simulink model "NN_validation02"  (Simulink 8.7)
settings: Solver=ode45  StartTime=0.0  StopTime=2000  RelTol=1e-3
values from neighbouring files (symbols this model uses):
  Ts = 0.2    [init_model.m]
libraries: neural x26

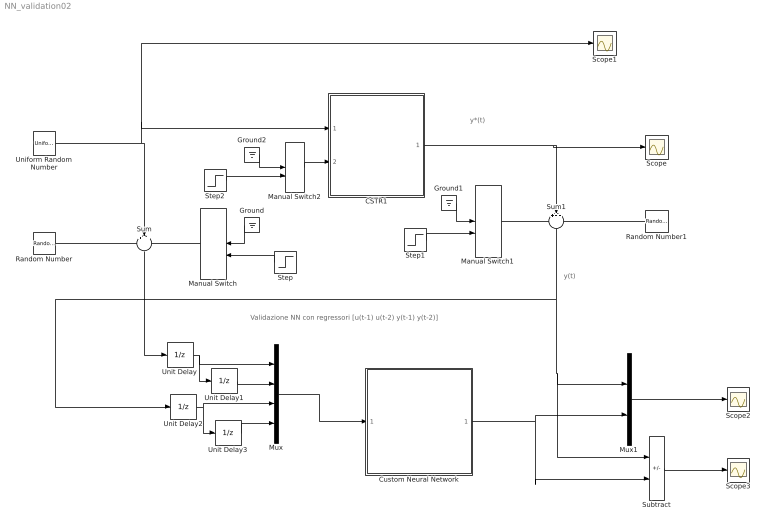
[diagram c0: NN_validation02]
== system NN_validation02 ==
  note: y(t)
  note: y*(t)
  note: Validazione NN con regressori [u(t-1) u(t-2) y(t-1) y(t-2)]
  CSTR1 : Subsystem
  Custom Neural Network : Subsystem
  Ground : Ground
  Ground1 : Ground
  Ground2 : Ground
  Manual Switch : ManualSwitch
  Manual Switch1 : ManualSwitch
  Manual Switch2 : ManualSwitch
  Mux : Mux
  Mux1 : Mux  Inputs=2
  Random Number : RandomNumber  Variance=0.0001  Seed=1  SampleTime=Ts
  Random Number1 : RandomNumber  Variance=0.0005  Seed=2  SampleTime=Ts
  Scope{,1..3} (4 alike) : Scope
  Step : Step  Time=1000  After=10  SampleTime=0
  Step1 : Step  Time=1000  After=10  SampleTime=0
  Step2 : Step  Time=1000  SampleTime=0
  Subtract : Sum  Inputs=+-
  Sum : Sum  Inputs=+++  SaturateOnIntegerOverflow=on
  Sum1 : Sum  Inputs=+++  SaturateOnIntegerOverflow=on
  Uniform Random Number : UniformRandomNumber  Minimum=0  Maximum=4  SampleTime=20
  Unit Delay{,1..3} (4 alike) : UnitDelay  SampleTime=Ts  HasFrameUpgradeWarning=on
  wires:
  Uniform Random Number/1 -> CSTR1/1(w), Scope1/1, Sum/2
  Random Number/1 -> Sum/1
  Manual Switch/1 -> Sum/3
  Sum/1 -> Unit Delay/1
  Ground/1 -> Manual Switch/1
  Step/1 -> Manual Switch/2
  Ground1/1 -> Manual Switch1/1
  Step1/1 -> Manual Switch1/2
  CSTR1/1(Cb) -> Scope/1, Sum1/2
  Manual Switch1/1 -> Sum1/1
  Random Number1/1 -> Sum1/3
  Unit Delay/1 -> Unit Delay1/1, Mux/1
  Unit Delay1/1 -> Mux/2
  Unit Delay2/1 -> Mux/3, Unit Delay3/1
  Unit Delay3/1 -> Mux/4
  Mux/1 -> Custom Neural Network/1(Input)
  Step2/1 -> Manual Switch2/2
  Manual Switch2/1 -> CSTR1/2(f)
  Ground2/1 -> Manual Switch2/1
  Subtract/1 -> Scope3/1
  Mux1/1 -> Scope2/1
  Sum1/1 -> Mux1/1, Subtract/1, Unit Delay2/1
  Custom Neural Network/1(Output) -> Subtract/2, Mux1/2

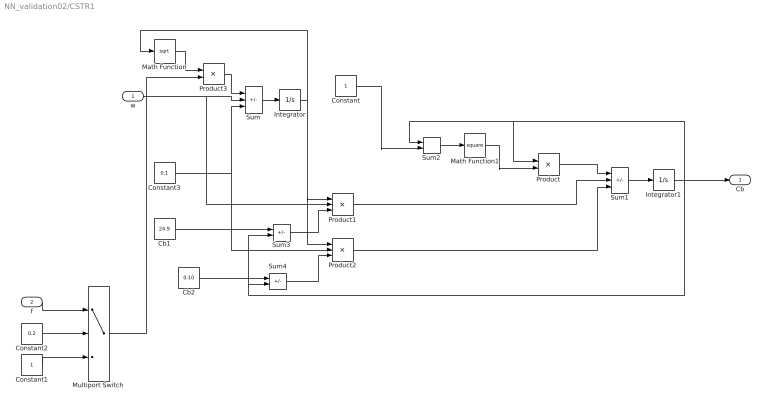
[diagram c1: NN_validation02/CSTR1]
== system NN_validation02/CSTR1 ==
  w : Inport
  f : Inport  Port=2
  Cb1 : Constant  Value=24.9
  Cb2 : Constant  Value=0.10
  Constant : Constant
  Constant1 : Constant
  Constant2 : Constant  Value=0.2
  Constant3 : Constant  Value=0.1
  Integrator : Integrator  InitialCondition=30  LimitOutput=on  LowerSaturationLimit=1
  Integrator1 : Integrator  InitialCondition=22
  Math Function : Math  Operator=sqrt
  Math Function1 : Math  Operator=square
  Multiport Switch : MultiPortSwitch  DataPortOrder=Zero-based contiguous  Inputs=2  zeroidx=on
  Product : Product  Inputs=*/  SaturateOnIntegerOverflow=on
  Product1 : Product  Inputs=/**  SaturateOnIntegerOverflow=on
  Product2 : Product  Inputs=/**  SaturateOnIntegerOverflow=on
  Product3 : Product
  Sum : Sum  Inputs=-++  SaturateOnIntegerOverflow=on
  Sum1 : Sum  Inputs=-++  SaturateOnIntegerOverflow=on
  Sum2 : Sum  SaturateOnIntegerOverflow=on
  Sum3 : Sum  Inputs=+-  SaturateOnIntegerOverflow=on
  Sum4 : Sum  Inputs=+-  SaturateOnIntegerOverflow=on
  Cb : Outport
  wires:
  Sum/1 -> Integrator/1
  Product3/1 -> Sum/1
  Math Function/1 -> Product3/1
  Integrator/1 -> Math Function/1, Product1/1, Product2/1
  Sum3/1 -> Product1/3
  Sum4/1 -> Product2/3
  Sum2/1 -> Math Function1/1
  Sum1/1 -> Integrator1/1
  Math Function1/1 -> Product/2
  Product/1 -> Sum1/1
  Product1/1 -> Sum1/2
  Product2/1 -> Sum1/3
  w/1 -> Sum/2, Product1/2
  Constant3/1 -> Product2/2, Sum/3
  Integrator1/1 -> Sum3/2, Sum4/2, Sum2/1, Product/1, Cb/1
  Constant1/1 -> Multiport Switch/3
  f/1 -> Multiport Switch/1
  Constant2/1 -> Multiport Switch/2
  Cb2/1 -> Sum4/1
  Cb1/1 -> Sum3/1
  Constant/1 -> Sum2/2
  Multiport Switch/1 -> Product3/2

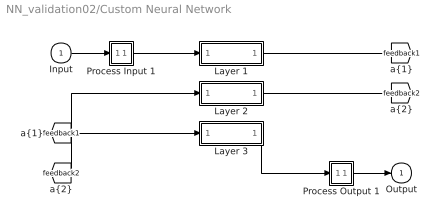
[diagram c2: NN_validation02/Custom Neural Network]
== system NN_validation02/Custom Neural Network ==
  Input : Inport  PortDimensions=4  SampleTime=0.2
  Layer 1 : Subsystem
  Layer 2 : Subsystem
  Layer 3 : Subsystem
  Process Input 1 : Subsystem
  Process Output 1 : Subsystem
  Output : Outport  InitialOutput=0
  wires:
  Input/1 -> Process Input 1/1(x)
  Process Output 1/1(y) -> Output/1
  Process Input 1/1(p) -> Layer 1/1("p{1}")
  Layer 1/1("a{1}") -> [feedback1]
  [feedback1] -> Layer 2/1("a{1} ")
  Layer 2/1("a{2}") -> [feedback2]
  [feedback2] -> Layer 3/1("a{2} ")
  Layer 3/1("a{3}") -> Process Output 1/1(a)

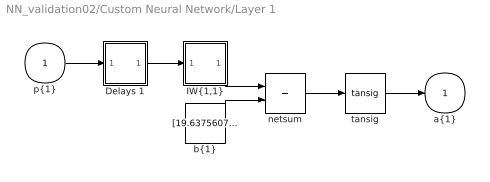
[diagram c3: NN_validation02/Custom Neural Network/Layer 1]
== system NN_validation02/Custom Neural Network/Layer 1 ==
  "p{1}" : Inport  PortDimensions=4  SampleTime=0.2
  Delays 1 : Subsystem
  "IW{1,1}" : Subsystem
  "b{1}" : Constant  Value=[19.637560791469059751079839770682156085968017578125;0.2047257682407544743252714170012040995061397552490234375;7.86074767430856535810335117275826632976531982421875;1.8383463614502668637129545459174551069736480712890625;-3.473396965964873128740464380825869739055633544921875;6.4026938213061885818433438544161617755889892578125;1.743354091492518964656710522831417620182037353515625]
  netsum : Sum  Inputs=2  InputSameDT=on  SaturateOnIntegerOverflow=on
  tansig : neural/Transfer Functions/tansig
  "a{1}" : Outport  InitialOutput=[0;0;0;0;0;0;0]
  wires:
  "p{1}"/1 -> Delays 1/1("p{1}")
  Delays 1/1("pd{1,1}") -> "IW{1,1}"/1("pd{1,1}")
  "IW{1,1}"/1("iz{1,1}") -> netsum/1
  "b{1}"/1 -> netsum/2
  netsum/1 -> tansig/1
  tansig/1 -> "a{1}"/1

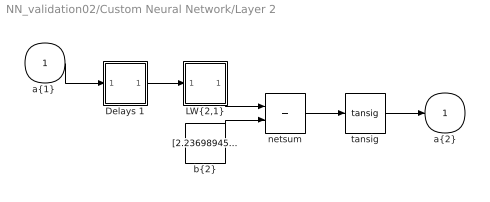
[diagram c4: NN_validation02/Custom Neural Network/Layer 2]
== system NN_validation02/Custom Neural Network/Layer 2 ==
  "a{1} " : Inport  PortDimensions=7  SampleTime=0.2
  Delays 1 : Subsystem
  "LW{2,1}" : Subsystem
  "b{2}" : Constant  Value=[2.23698945546536887007960103801451623439788818359375;3.791807829950591735013176730717532336711883544921875;-3.050918615819495638419311944744549691677093505859375;1.458459391661695914166330112493596971035003662109375;-0.26735871458239468534401339638861827552318572998046875;-3.409507071588366411418746793060563504695892333984375;4.58163129532917157149540798855014145374298095703125;1.1083081740108098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
  netsum : Sum  Inputs=2  InputSameDT=on  SaturateOnIntegerOverflow=on
  tansig : neural/Transfer Functions/tansig
  "a{2}" : Outport  InitialOutput=[0;0;0;0;0;0;0;0;0;0;0;0;0;0;0]
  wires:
  "a{1} "/1 -> Delays 1/1("p{2}")
  Delays 1/1("pd{2,1}") -> "LW{2,1}"/1("ad{2,1}")
  "LW{2,1}"/1("lz{2,1}") -> netsum/1
  "b{2}"/1 -> netsum/2
  netsum/1 -> tansig/1
  tansig/1 -> "a{2}"/1

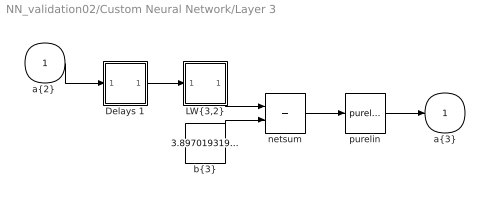
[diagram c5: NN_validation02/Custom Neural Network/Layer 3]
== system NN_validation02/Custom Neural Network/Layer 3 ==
  "a{2} " : Inport  PortDimensions=15  SampleTime=0.2
  Delays 1 : Subsystem
  "LW{3,2}" : Subsystem
  "b{3}" : Constant  Value=3.897019319091107103503190955962054431438446044921875
  netsum : Sum  Inputs=2  InputSameDT=on  SaturateOnIntegerOverflow=on
  purelin : neural/Transfer Functions/purelin
  "a{3}" : Outport  InitialOutput=0
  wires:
  "a{2} "/1 -> Delays 1/1("p{3}")
  Delays 1/1("pd{3,2}") -> "LW{3,2}"/1("ad{3,2}")
  "LW{3,2}"/1("lz{3,2}") -> netsum/1
  "b{3}"/1 -> netsum/2
  netsum/1 -> purelin/1
  purelin/1 -> "a{3}"/1

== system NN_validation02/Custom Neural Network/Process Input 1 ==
  x : Inport  PortDimensions=4  SampleTime=0.2
  p : Outport  PortDimensions=4  SampleTime=0.2
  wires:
  x/1 -> p/1

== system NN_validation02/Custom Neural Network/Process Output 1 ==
  a : Inport  PortDimensions=1  SampleTime=0.2
  y : Outport  PortDimensions=1  SampleTime=0.2
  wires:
  a/1 -> y/1

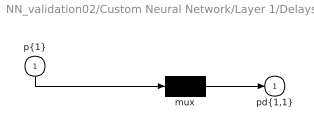
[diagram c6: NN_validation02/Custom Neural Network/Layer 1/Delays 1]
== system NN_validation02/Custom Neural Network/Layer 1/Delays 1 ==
  "p{1}" : Inport  PortDimensions=4  SampleTime=0.2
  mux : Mux  Inputs=1
  "pd{1,1}" : Outport
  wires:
  "p{1}"/1 -> mux/1
  mux/1 -> "pd{1,1}"/1

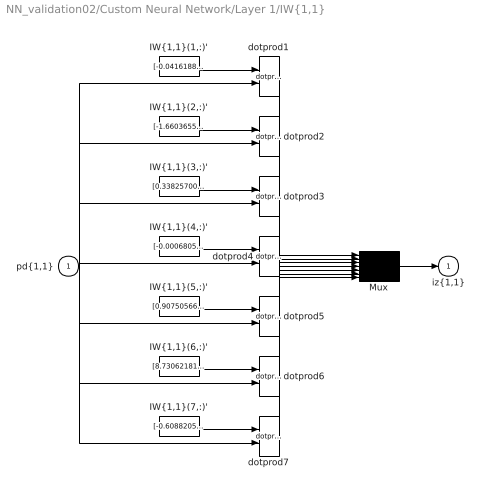
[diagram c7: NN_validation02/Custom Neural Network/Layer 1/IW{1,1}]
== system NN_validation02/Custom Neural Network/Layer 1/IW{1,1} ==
  "pd{1,1}" : Inport  PortDimensions=4  SampleTime=0.2
  "IW{1,1}(1,:)'" : Constant  Value=[-0.041618886227972252955797927143066772259771823883056640625;-0.73919056812561068081635085036396048963069915771484375;-1.4422835941292893036091982139623723924160003662109375;0.04139514251946392608960678671792265959084033966064453125]
  "IW{1,1}(2,:)'" : Constant  Value=[-1.6603655645525836614950776493060402572154998779296875;-3.905595226797782704153405575198121368885040283203125;2.157699450980562705382226340589113533496856689453125;-0.2448018441202345629736925047836848534643650054931640625]
  "IW{1,1}(3,:)'" : Constant  Value=[0.3382570022825082123318907179054804146289825439453125;-12.430785938215979768983743269927799701690673828125;0.8764590009724495534015886732959188520908355712890625;-1.3683079527560604304881053394638001918792724609375]
  "IW{1,1}(4,:)'" : Constant  Value=[-0.00068051177936000466391075480743211301160044968128204345703125;5.8527872840413827822125814037690361146815121173858642578125e-05;-0.05975031240672733223728840812327689491212368011474609375;-0.048301987882430709453362993599512265063822269439697265625]
  "IW{1,1}(5,:)'" : Constant  Value=[0.90750566248841069150188332059769891202449798583984375;2.450597393074088525821707662544213235378265380859375;0.5711269731156882745182201688294298946857452392578125;0.4443580313075894405727694902452640235424041748046875]
  "IW{1,1}(6,:)'" : Constant  Value=[8.730621815224044013348247972317039966583251953125;10.231045364355342286444283672608435153961181640625;-0.9152993340520854115283100327360443770885467529296875;-0.041852906712550208556677944216062314808368682861328125]
  "IW{1,1}(7,:)'" : Constant  Value=[-0.60882051341333187632898216179455630481243133544921875;-0.066422912329109184970121759761241264641284942626953125;0.613340824515325788723885125364176928997039794921875;-0.09785652025840875511963901089984574355185031890869140625]
  Mux : Mux  Inputs=7
  dotprod{1..7} (7 alike) : neural/Weight Functions/dotprod
  "iz{1,1}" : Outport
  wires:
  "IW{1,1}(1,:)'"/1 -> dotprod1/1
  "pd{1,1}"/1 -> dotprod1/2, dotprod2/2, dotprod3/2, dotprod4/2, dotprod5/2, dotprod6/2, dotprod7/2
  dotprod1/1 -> Mux/1
  "IW{1,1}(2,:)'"/1 -> dotprod2/1
  dotprod2/1 -> Mux/2
  "IW{1,1}(3,:)'"/1 -> dotprod3/1
  dotprod3/1 -> Mux/3
  "IW{1,1}(4,:)'"/1 -> dotprod4/1
  dotprod4/1 -> Mux/4
  "IW{1,1}(5,:)'"/1 -> dotprod5/1
  dotprod5/1 -> Mux/5
  "IW{1,1}(6,:)'"/1 -> dotprod6/1
  dotprod6/1 -> Mux/6
  "IW{1,1}(7,:)'"/1 -> dotprod7/1
  dotprod7/1 -> Mux/7
  Mux/1 -> "iz{1,1}"/1

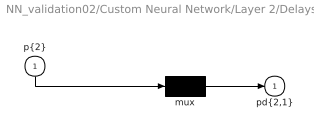
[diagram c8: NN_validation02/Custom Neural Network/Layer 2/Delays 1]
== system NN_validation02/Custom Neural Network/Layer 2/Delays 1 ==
  "p{2}" : Inport  PortDimensions=7  SampleTime=0.2
  mux : Mux  Inputs=1
  "pd{2,1}" : Outport
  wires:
  "p{2}"/1 -> mux/1
  mux/1 -> "pd{2,1}"/1

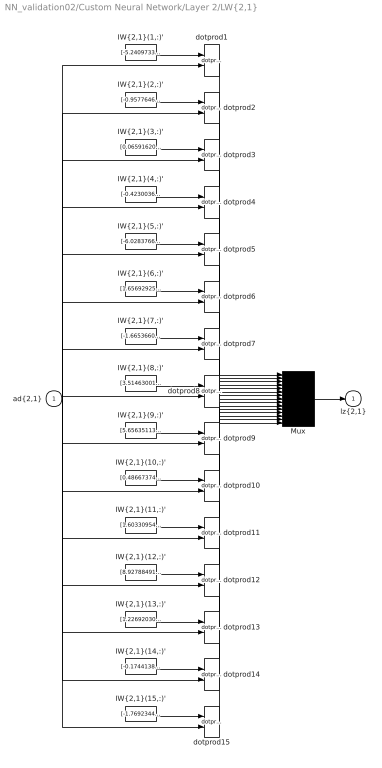
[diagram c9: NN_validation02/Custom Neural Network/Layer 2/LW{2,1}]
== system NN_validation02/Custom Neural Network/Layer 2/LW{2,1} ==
  "ad{2,1}" : Inport  PortDimensions=7  SampleTime=0.2
  "IW{2,1}(1,:)'" : Constant  Value=[-5.2409733372715567867317076888866722583770751953125;-0.23294355714330616802243412166717462241649627685546875;2.18290533615787563093135759118013083934783935546875;4.5111511516424531720304003101773560047149658203125;0.712098578582030850014916723011992871761322021484375;-8.1542869471625198940500922617502510547637939453125;-1.0643885537349053738154225356993265450000762939453125]
  "IW{2,1}(10,:)'" : Constant  Value=[0.486673743874140918297399593939189799129962921142578125;-0.8445116995008909999143043023650534451007843017578125;1.0027984302568970775837442488409578800201416015625;-0.10413427371086696193724918657608213834464550018310546875;0.2105384193571350481821724542896845377981662750244140625;3.13524741281104724066608469001948833465576171875;0.8974294333879069274217954443884082138538360595703125]
  "IW{2,1}(11,:)'" : Constant  Value=[1.60330954272756809331212934921495616436004638671875;-0.271718628322324351476169113084324635565280914306640625;-0.82920303789284532935965899014263413846492767333984375;-2.540460142238908591849622098379768431186676025390625;-1.1466434528964495331848638670635409653186798095703125;0.024493350163058709434427129281175439245998859405517578125;-0.7129096923507212135717736600781790912151336669921875]
  "IW{2,1}(12,:)'" : Constant  Value=[8.927884919836476029786354047246277332305908203125;-1.007332576938406276667592464946210384368896484375;1.2685489106433376349514219327829778194427490234375;7.907882070121072359825120656751096248626708984375;-1.8242100818082327418068189217592589557170867919921875;-2.71824423482211496860827537602744996547698974609375;-0.25767480325555591758046602990361861884593963623046875]
  "IW{2,1}(13,:)'" : Constant  Value=[1.2269203094374152573919900532928295433521270751953125;0.248350582057697388815853400956257246434688568115234375;-0.5079254295367743310407604440115392208099365234375;-0.1901720937384543674841808069686521776020526885986328125;1.8066997392792087939739076318801380693912506103515625;0.343192072589101171420367109021754004061222076416015625;1.117282779665665248813866128330118954181671142578125]
  "IW{2,1}(14,:)'" : Constant  Value=[-0.174413863339862473811336940343608148396015167236328125;-0.34807694820884427233664837331161834299564361572265625;0.437718162177463010475975124791148118674755096435546875;-1.314962655193088636451648198999464511871337890625;-2.316860450083221945050127033027820289134979248046875;-0.68727152283431058865659224466071464121341705322265625;-0.32864666867050329468469271887443028390407562255859375]
  "IW{2,1}(15,:)'" : Constant  Value=[-1.7692344875232997036818005653913132846355438232421875;2.606315815077001385446919812238775193691253662109375;-1.294710238055885032082414909382350742816925048828125;2.06504745193336791686533615575172007083892822265625;2.98426857853844840207102606655098497867584228515625;-0.70826881977382782906715874560177326202392578125;2.709113982711269574821244532358832657337188720703125]
  "IW{2,1}(2,:)'" : Constant  Value=[-0.95776462082827651389749235022463835775852203369140625;-0.75046016315013108766152072348631918430328369140625;-0.71751895609824767330309214230510406196117401123046875;-0.379935303078497599305052290219464339315891265869140625;1.4060950432554670808116270563914440572261810302734375;0.724418683520327011393646898795850574970245361328125;1.28975634466395394639448568341322243213653564453125]
  "IW{2,1}(3,:)'" : Constant  Value=[0.06591620278996547510619308241075486876070499420166015625;-1.2750459834710186068917892043828032910823822021484375;0.00951003700790489965577467756929763709194958209991455078125;-0.0676443119919310775767229415578185580670833587646484375;-0.67359886701772653250230860066949389874935150146484375;0.09184816025641782955002412336398265324532985687255859375;0.026201338814941851212969581297329568769782781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
  "IW{2,1}(4,:)'" : Constant  Value=[-0.423003684813168467915289738812134601175785064697265625;1.94165248913885957193770082085393369197845458984375;-0.4214309658599233454623345096479170024394989013671875;0.421440321829336828063361508611706085503101348876953125;1.134787536819579667479729323531500995159149169921875;0.64734269121063847673980262698023580014705657958984375;1.7441643434793372424707058598869480192661285400390625]
  "IW{2,1}(5,:)'" : Constant  Value=[-6.02837665862743232736420395667664706707000732421875;-0.827772995089444574290382661274634301662445068359375;2.488678578524841089603114596684463322162628173828125;9.0553682810267712710583509760908782482147216796875;-1.323392759528513096256574499420821666717529296875;-2.16624194768094024965421340311877429485321044921875;-0.95423270177042740503026152509846724569797515869140625]
  "IW{2,1}(6,:)'" : Constant  Value=[1.6569292594035525123530305791064165532588958740234375;-3.700197161529342526620212083798833191394805908203125;-0.55081165507598850439308080240152776241302490234375;3.152522214052721150068236966035328805446624755859375;-5.52774929656755542595192309818230569362640380859375;-5.7080344103869382621496697538532316684722900390625;-5.08326678775291096457067396841011941432952880859375]
  "IW{2,1}(7,:)'" : Constant  Value=[-1.665366018786639035198504643631167709827423095703125;4.8024434195461314089925508596934378147125244140625;-0.88480189609406867390362094738520681858062744140625;4.01813497507322114898897780221886932849884033203125;4.17705320201275043245914275757968425750732421875;-0.54173322595133155399338420465937815606594085693359375;3.90493751644229636355021284543909132480621337890625]
  "IW{2,1}(8,:)'" : Constant  Value=[3.514630016714414662004628553404472768306732177734375;0.6581198867674469266120240718009881675243377685546875;-3.548815874605704578925724490545690059661865234375;7.47429102799332412132571334950625896453857421875;0.0747477198151732802333668814753764308989048004150390625;3.46581469752752280300001075374893844127655029296875;2.14906571991818662326068078982643783092498779296875]
  "IW{2,1}(9,:)'" : Constant  Value=[5.65635113578725867711227692780084908008575439453125;0.350214830981460056857912377381580881774425506591796875;0.9507107352465331562285655309096910059452056884765625;1.0772243986264740112090976253966800868511199951171875;0.18288157186065656656381861466798000037670135498046875;3.272197921136366094430059092701412737369537353515625;-0.51173914238865503278930191299878060817718505859375]
  Mux : Mux  Inputs=15
  dotprod{1..15} (15 alike) : neural/Weight Functions/dotprod
  "lz{2,1}" : Outport
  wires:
  "IW{2,1}(1,:)'"/1 -> dotprod1/1
  "ad{2,1}"/1 -> dotprod1/2, dotprod2/2, dotprod3/2, dotprod4/2, dotprod5/2, dotprod6/2, dotprod7/2, dotprod8/2, dotprod9/2, dotprod10/2, dotprod11/2, dotprod12/2, dotprod13/2, dotprod14/2, dotprod15/2
  dotprod1/1 -> Mux/1
  "IW{2,1}(2,:)'"/1 -> dotprod2/1
  dotprod2/1 -> Mux/2
  "IW{2,1}(3,:)'"/1 -> dotprod3/1
  dotprod3/1 -> Mux/3
  "IW{2,1}(4,:)'"/1 -> dotprod4/1
  dotprod4/1 -> Mux/4
  "IW{2,1}(5,:)'"/1 -> dotprod5/1
  dotprod5/1 -> Mux/5
  "IW{2,1}(6,:)'"/1 -> dotprod6/1
  dotprod6/1 -> Mux/6
  "IW{2,1}(7,:)'"/1 -> dotprod7/1
  dotprod7/1 -> Mux/7
  "IW{2,1}(8,:)'"/1 -> dotprod8/1
  dotprod8/1 -> Mux/8
  "IW{2,1}(9,:)'"/1 -> dotprod9/1
  dotprod9/1 -> Mux/9
  "IW{2,1}(10,:)'"/1 -> dotprod10/1
  dotprod10/1 -> Mux/10
  "IW{2,1}(11,:)'"/1 -> dotprod11/1
  dotprod11/1 -> Mux/11
  "IW{2,1}(12,:)'"/1 -> dotprod12/1
  dotprod12/1 -> Mux/12
  "IW{2,1}(13,:)'"/1 -> dotprod13/1
  dotprod13/1 -> Mux/13
  "IW{2,1}(14,:)'"/1 -> dotprod14/1
  dotprod14/1 -> Mux/14
  "IW{2,1}(15,:)'"/1 -> dotprod15/1
  dotprod15/1 -> Mux/15
  Mux/1 -> "lz{2,1}"/1

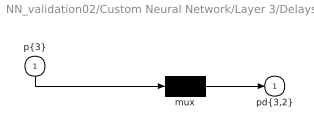
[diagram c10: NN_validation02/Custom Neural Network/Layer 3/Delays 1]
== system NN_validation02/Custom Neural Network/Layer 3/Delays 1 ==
  "p{3}" : Inport  PortDimensions=15  SampleTime=0.2
  mux : Mux  Inputs=1
  "pd{3,2}" : Outport
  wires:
  "p{3}"/1 -> mux/1
  mux/1 -> "pd{3,2}"/1

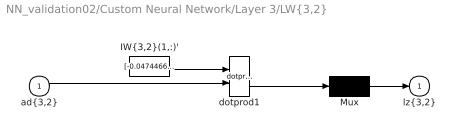
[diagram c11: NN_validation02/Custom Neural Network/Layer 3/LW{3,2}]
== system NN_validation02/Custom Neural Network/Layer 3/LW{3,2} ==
  "ad{3,2}" : Inport  PortDimensions=15  SampleTime=0.2
  "IW{3,2}(1,:)'" : Constant  Value=[-0.04744668366631221712026444947696290910243988037109375;2.042401955341885066985696539632044732570648193359375;-0.258399104803635315530385696547455154359340667724609375;2.908429506539129238973373503540642559528350830078125;-0.102740019563529683122027336139581166207790374755859375;-1.3874079538647146048191416412009857594966888427734375;-2.069729771701947829143364288029260933399200439453125;-0.0933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
  Mux : Mux  Inputs=1
  dotprod1 : neural/Weight Functions/dotprod
  "lz{3,2}" : Outport
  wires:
  "IW{3,2}(1,:)'"/1 -> dotprod1/1
  "ad{3,2}"/1 -> dotprod1/2
  dotprod1/1 -> Mux/1
  Mux/1 -> "lz{3,2}"/1
